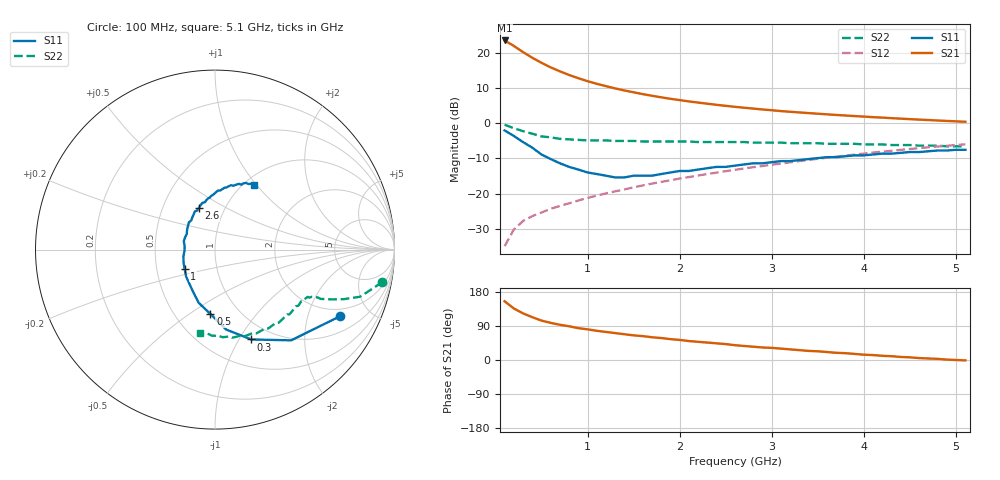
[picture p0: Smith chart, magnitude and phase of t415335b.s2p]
!AT-41533
!S and NOISE PARAMETERS at Vce=5V Ic=5mA. LAST UPDATED 01-25-95
# ghz s ma r 50
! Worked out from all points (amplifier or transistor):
!   51 points, 100 MHz to 5.1 GHz, reference 50 ohm
!   highest |S21| = 23.5 dB at 100 MHz (marker M1)
!   |S21| within 3 dB of that: start of sweep to 283.1 MHz
!   unconditionally stable (mu >= 1): 908.2 MHz to 2.357 GHz
!   at 900 MHz: K = 1.00, MSG = 17.4 dB, |S12| = -21.9 dB
!   at 2.6 GHz: K = 0.97, MSG = 8.9 dB, |S12| = -13.2 dB
!   at 5.1 GHz: K = 0.83, MSG = 3.2 dB, |S12| = -6.0 dB
!   lowest NFmin = 0.70 dB at 100 MHz
!   S11 on the Smith chart (normalised r, x): 100 MHz: 1.64, -3.24; 300 MHz: 0.80, -1.13; 500 MHz: 0.74, -0.61; 1 GHz: 0.70, -0.15; 2.6 GHz: 0.76, +0.38; 5.1 GHz: 1.11, +0.97
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0.1  0.79 -28.0  14.93 155.0  0.018 76.0  0.95 -11.0
0.2  0.66 -50.0  12.49 136.0  0.031 67.0  0.85 -18.0
0.3  0.54 -68.0  10.22 123.0  0.041 63.0  0.77 -21.0
0.4  0.45 -82.0  8.49 113.0  0.048 61.0  0.71 -23.0
0.5  0.36 -94.0  7.2 104.0  0.054 61.0  0.65 -25.0
0.6  0.31 -107.0  6.199 98.0  0.061 61.0  0.63 -25.0
0.7  0.27 -116.0  5.446 93.0  0.067 62.0  0.6 -26.0
0.8  0.24 -126.0  4.832 89.0  0.073 63.0  0.59 -27.0
0.9  0.22 -137.0  4.349 84.0  0.08 63.0  0.58 -27.0
1  0.2 -148.0  3.948 81.0  0.087 64.0  0.57 -29.0
1.1  0.19 -157.0  3.624 77.0  0.094 65.0  0.57 -29.0
1.3  0.17 -178.0  3.116 71.0  0.108 65.0  0.56 -31.0
1.4  0.17 174.0  2.915 68.0  0.115 65.0  0.56 -32.0
1.7  0.18 151.0  2.45 60.0  0.139 65.0  0.55 -36.0
1.8  0.19 145.0  2.328 58.0  0.147 65.0  0.55 -37.0
2.1  0.21 129.0  2.037 50.0  0.172 64.0  0.55 -41.0
2.6  0.25 111.0  1.708 39.0  0.218 62.0  0.54 -48.0
2.9  0.27 102.0  1.566 33.0  0.247 60.0  0.53 -53.0
3.5  0.32 89.0  1.363 23.0  0.313 55.0  0.52 -64.0
4  0.35 80.0  1.24 14.0  0.371 50.0  0.5 -74.0
4.3  0.37 74.0  1.179 10.0  0.406 46.0  0.49 -81.0
5.1  0.42 59.0  1.048 -1.0  0.502 36.0  0.47 -100.0
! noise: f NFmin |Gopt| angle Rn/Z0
0.1  0.7  0.46  7  0.21
0.9  1  0.29  86  0.13
1.8  1.4  0.36  -163  0.07
2.4  1.6  0.53  -127  0.15
